TYPE ST_SlaveState :
STRUCT
	(* slave state *)
	eEcState 		: E_EcCommState;
	nReserved		: UINT;
	bError			: BOOL;
	bInvalidVPRS	: BOOL;
	nReserved2		: UINT;

	(* link state *)
	bNoCommToSlave	: BOOL;
	bLinkError		: BOOL;
	bMissingLink	: BOOL;
	bUnexpectedLink	: BOOL;
	bPortA			: BOOL;
	bPortB			: BOOL;
	bPortC			: BOOL;
	bPortD			: BOOL;
END_STRUCT
END_TYPE
